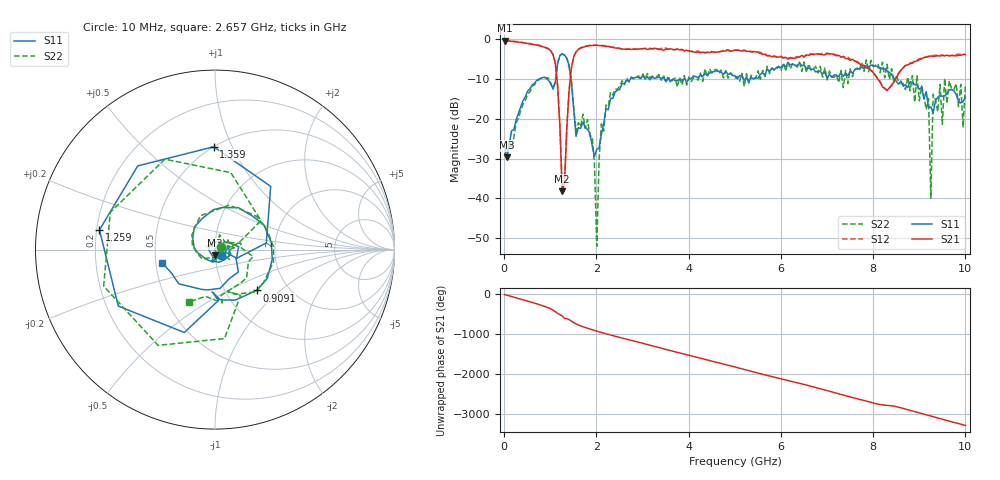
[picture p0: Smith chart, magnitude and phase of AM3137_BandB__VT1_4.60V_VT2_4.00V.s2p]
! Date/Time: Tue, Nov 13, 2018 4:52 PM
! Network Analyzer: Agilent Technologies E8364B Rev: A.07.50.67
! Sweep from 0.010 to 10.000 GHz, 201 Points, Sweep Type: LIN
! Power Supply: 4.601 V, 0.002 A
# Hz S DB R 50
!freq MagS11 AngS11 MagS21 AngS21 MagS12 AngS12 MagS22 AngS22
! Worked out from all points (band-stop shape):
!   201 points, 10 MHz to 10 GHz, reference 50 ohm
!   highest |S21| = -0.36 dB at 10 MHz (marker M1); lowest = -38.2 dB at 1.259 GHz (marker M2)
!   |S21| within 3 dB of the highest: 1.554 GHz to 4.235 GHz (2.682 GHz wide, 92.7 % of centre); 4.467 GHz to 5.512 GHz (1.045 GHz wide, 20.9 % of centre)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
!   lowest |S11| = -29.7 dB at 59.95 MHz (marker M3), VSWR 1.07, Z = 49.8 - j3.26 ohm
!   |S11| at or under -10 dB: start of sweep to 758.9 MHz; 1.449 GHz to 2.739 GHz (1.29 GHz wide, 61.6 % of centre); 8.461 GHz to end of sweep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
!   |S22| runs from -52.0 to -3.7 dB; largest |S21 - S12| = 0.042
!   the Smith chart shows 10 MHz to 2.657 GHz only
!   S11 on the Smith chart (normalised r, x): 10 MHz: 1.07, -0.06; 909.1 MHz: 1.39, -0.71; 1.259 GHz: 0.21, +0.08; 1.359 GHz: 0.50, +0.85; 2.657 GHz: 0.54, -0.09
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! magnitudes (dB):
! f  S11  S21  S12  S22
! 10 MHz  -26.8  -0.4  -0.3  -28.6
! 59.95 MHz  -29.7  -0.4  -0.3  -29.7
! 909.1 MHz  -9.8  -2.2  -2.1  -9.7
! 1.109 GHz  -10.9  -6.1  -6.0  -10.7
! 1.259 GHz  -3.7  -38.2  -38.0  -3.7
! 1.359 GHz  -4.8  -22.2  -22.3  -4.8
! 1.558 GHz  -24.4  -3.2  -3.2  -23.1
! 1.708 GHz  -20.8  -2.1  -2.0  -18.8
! 1.908 GHz  -26.7  -1.6  -1.5  -24.4
! 2.008 GHz  -27.7  -1.6  -1.5  -52.0
! 2.108 GHz  -23.9  -1.7  -1.6  -21.3
! 2.657 GHz  -10.4  -2.6  -2.5  -9.8
! 3.357 GHz  -9.5  -2.6  -2.5  -8.9
! 5.005 GHz  -9.2  -2.8  -2.8  -9.8
! 6.703 GHz  -7.5  -3.9  -3.7  -7.5
! 8.352 GHz  -8.4  -12.2  -12.3  -10.1
! 9.201 GHz  -17.2  -4.3  -4.4  -14.9
! 9.251 GHz  -17.0  -4.2  -4.2  -39.9
! 9.301 GHz  -18.6  -4.3  -4.1  -13.8
! 9.9 GHz  -16.0  -4.1  -3.9  -11.4
! 9.95 GHz  -15.7  -3.9  -3.8  -22.0
! 10 GHz  -14.6  -3.9  -3.8  -11.6
